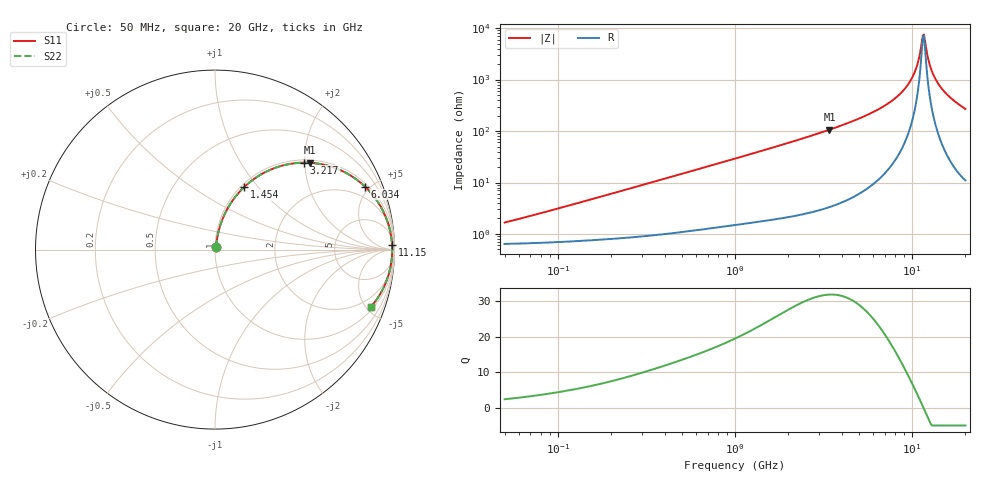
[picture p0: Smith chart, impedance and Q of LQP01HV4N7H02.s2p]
!Murata Part Number: LQP01HV4N7H02
!These Parameters are Measured in Series Mode Connection
!  o--[Z]--o
!Port1  Port2
!  o-------o
!Freq. Start=50[MHz] Stop=20[GHz], 401[Steps]
# Hz S RI R 50
!Freq.(Hz) S11(Real) S11(Imag) S21(Real) S21(Imag) S12(Real) S12(Imag) S22(Real) S22(Imag)
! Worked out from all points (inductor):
!   401 points, 50 MHz to 20 GHz, reference 50 ohm
!   read as one part in series: L = 4.87 nH near 64.5 MHz
!   highest Q = 31.9 at 3.415 GHz (marker M1), where L = 4.95 nH
!   self-resonance near 11.49 GHz
!   S11 on the Smith chart (normalised r, x): 50 MHz: 1.01, +0.03; 1.454 GHz: 1.04, +0.85; 3.217 GHz: 1.06, +1.98; 6.034 GHz: 1.19, +4.68; 11.15 GHz: 35, +64; 20 GHz: 1.22, -5.38
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5e7  0.0066 0.0152  0.9934 -0.0152  0.9934 -0.0152  0.0066 0.0152
1.364002e8  0.00897 0.0406  0.991 -0.0406  0.991 -0.0406  0.00897 0.0406
3.721004e8  0.0212 0.1067  0.9788 -0.1067  0.9788 -0.1067  0.0212 0.1067
1e9  0.0895 0.2611  0.9105 -0.2611  0.9105 -0.2611  0.0895 0.2611
1.454215e9  0.1627 0.3486  0.8373 -0.3486  0.8373 -0.3486  0.1627 0.3486
2.728004e9  0.4065 0.4753  0.5935 -0.4753  0.5935 -0.4753  0.4065 0.4753
3.216634e9  0.4957 0.4845  0.5043 -0.4845  0.5043 -0.4845  0.4957 0.4845
3.415248e9  0.5296 0.4837  0.4704 -0.4837  0.4704 -0.4837  0.5296 0.4837
6.034176e9  0.8361 0.3508  0.1639 -0.3508  0.1639 -0.3508  0.8361 0.3508
7.442007e9  0.9157 0.2523  0.0843 -0.2523  0.0843 -0.2523  0.9157 0.2523
8.644534e9  0.9553 0.1718  0.0447 -0.1718  0.0447 -0.1718  0.9553 0.1718
9.745021e9  0.9758 0.1033  0.0242 -0.1033  0.0242 -0.1033  0.9758 0.1033
1.050288e10  0.9835 0.0593  0.0165 -0.0593  0.0165 -0.0593  0.9835 0.0593
1.082228e10  0.9854 0.0415  0.0146 -0.0415  0.0146 -0.0415  0.9854 0.0415
1.115139e10  0.9866 0.0236  0.0134 -0.0236  0.0134 -0.0236  0.9866 0.0236
1.149051e10  0.9873 0.0057  0.0127 -0.0057  0.0127 -0.0057  0.9873 0.0057
1.166392e10  0.9873 -0.00328  0.0127 0.00328  0.0127 0.00328  0.9873 -0.00328
1.183995e10  0.9872 -0.0123  0.0128 0.0123  0.0128 0.0123  0.9872 -0.0123
1.276073e10  0.9841 -0.0573  0.0159 0.0573  0.0159 0.0573  0.9841 -0.0573
1.396067e10  0.9748 -0.1112  0.0252 0.1112  0.0252 0.1112  0.9748 -0.1112
1.621653e10  0.9451 -0.1996  0.0549 0.1996  0.0549 0.1996  0.9451 -0.1996
2e10  0.8688 -0.3177  0.1312 0.3177  0.1312 0.3177  0.8688 -0.3177
